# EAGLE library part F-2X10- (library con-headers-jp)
FEMALE HEADER
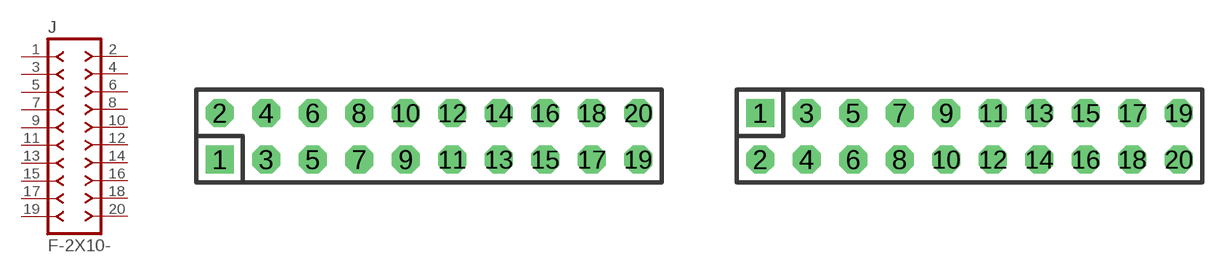
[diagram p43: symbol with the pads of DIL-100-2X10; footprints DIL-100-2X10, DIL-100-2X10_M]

Designator prefix J

## F-2X10-DIL-100  [DIL-100-2X10]
1  1  pas
2  2  pas
3  3  pas
4  4  pas
5  5  pas
6  6  pas
7  7  pas
8  8  pas
9  9  pas
10  10  pas
11  11  pas
12  12  pas
13  13  pas
14  14  pas
15  15  pas
16  16  pas
17  17  pas
18  18  pas
19  19  pas
20  20  pas

## F-2X10-DIL-100_M  [DIL-100-2X10_M]
Pads as for DIL-100-2X10

## F-2X10-DIL-2MM  [DIL-2MM-2X10]
Pads as for DIL-100-2X10

## F-2X10-DIL-2MM_M  [DIL-2MM-2X10_M]
Pads as for DIL-100-2X10

## F-2X10-71991  [71991-20]
Pads as for DIL-100-2X10

## F-2X10-79107  [79107-20]
Pads as for DIL-100-2X10

## F-2X10-79107_M  [79107-20_M]
Pads as for DIL-100-2X10

## Footprint DIL-100-2X10 (pad centres in mm)
PIN HEADER - 0.1"
drill 1.016 square: 1 -11.43,-1.27
drill 1.016 octagon: 2 -11.43,1.27; 3 -8.89,-1.27; 4 -8.89,1.27; 5 -6.35,-1.27; 6 -6.35,1.27; 7 -3.81,-1.27; 8 -3.81,1.27; 9 -1.27,-1.27; 10 -1.27,1.27; 11 1.27,-1.27; 12 1.27,1.27; 13 3.81,-1.27; 14 3.81,1.27; 15 6.35,-1.27; 16 6.35,1.27; 17 8.89,-1.27; 18 8.89,1.27; 19 11.43,-1.27; 20 11.43,1.27

## Footprint DIL-100-2X10_M (pad centres in mm)
PIN HEADER - MIRRORED 0.1"
drill 1.016 square: 1 -11.43,1.27
drill 1.016 octagon: 2 -11.43,-1.27; 3 -8.89,1.27; 4 -8.89,-1.27; 5 -6.35,1.27; 6 -6.35,-1.27; 7 -3.81,1.27; 8 -3.81,-1.27; 9 -1.27,1.27; 10 -1.27,-1.27; 11 1.27,1.27; 12 1.27,-1.27; 13 3.81,1.27; 14 3.81,-1.27; 15 6.35,1.27; 16 6.35,-1.27; 17 8.89,1.27; 18 8.89,-1.27; 19 11.43,1.27; 20 11.43,-1.27

## Footprint DIL-2MM-2X10 (pad centres in mm)
PIN HEADER - 2MM"
drill 0.711 square: 1 -9,-1
drill 0.711: 2 -9,1; 3 -7,-1; 4 -7,1; 5 -5,-1; 6 -5,1; 7 -3,-1; 8 -3,1; 9 -1,-1; 10 -1,1; 11 1,-1; 12 1,1; 13 3,-1; 14 3,1; 15 5,-1; 16 5,1; 17 7,-1; 18 7,1; 19 9,-1; 20 9,1

## Footprint DIL-2MM-2X10_M (pad centres in mm)
PIN HEADER - MIRRORED 2MM
drill 0.711 square: 1 -9,1
drill 0.711: 2 -9,-1; 3 -7,1; 4 -7,-1; 5 -5,1; 6 -5,-1; 7 -3,1; 8 -3,-1; 9 -1,1; 10 -1,-1; 11 1,1; 12 1,-1; 13 3,1; 14 3,-1; 15 5,1; 16 5,-1; 17 7,1; 18 7,-1; 19 9,1; 20 9,-1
